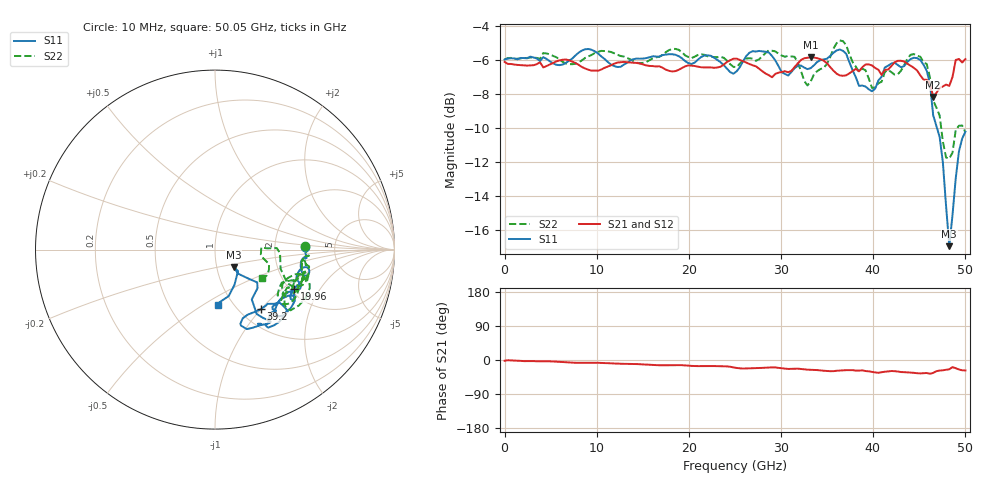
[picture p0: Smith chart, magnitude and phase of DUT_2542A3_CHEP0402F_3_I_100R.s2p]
! 11/3/2025 4:29:20 PM
! C:\MESURES\046-TRL-DUT-CHEP\0402\DUT-2542A3-CHEP0402F-3-I.S2P
! CHANNEL.1 Sparams
! TR.MEASUREMENT
! CORRECTED.DATA
! RF.CORRECTION: CAL.A: FULL.TWO.PORT.CALCAL.A: Port 1,4
! AVERAGING.OFF
! IF.BANDWIDTH: 500HZ
! SWEEPTYPE:  FREQ.SWEEP(Linear)
! Reference Plane Port Info
! PORT:  PORT1  PORT4
! DISTANCE:  0  m  0  m
! TIME:  0  s  0  s
! PHASE.OFFSET:  0  deg.  0  deg.
! LOSS:  0  dB  0  dB
! REF.LOSS:  0  dB  0  dB
! REF.FREQ:  0  Hz  0  Hz
! Power Info
! POWER:  -10  dBm  -10  dBm
! EFF.POWER:  -10  dBm  -10  dBm
! SOURCE.ATTEN:  0  dB  0  dB
! TEST.ATTEN:  0  dB  0  dB
! PORTZ: Port1:50 Port4:50
# GHZ S RI R 50
! FREQ.GHZ  S11RE  S11IM  S41RE  S41IM  S14RE  S14IM  S44RE  S44IM
!; PortSelection: Port_14 (1-->1,4-->4)
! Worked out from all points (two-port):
!   144 points, 10 MHz to 50.05 GHz, reference 50 ohm
!   highest |S21| = -5.84 dB at 33.26 GHz (marker M1); lowest = -8.2 dB at 46.55 GHz (marker M2)
!   |S21| within 3 dB of the highest: start of sweep to end of sweep
!   lowest |S11| = -17.0 dB at 48.3 GHz (marker M3), VSWR 1.33, Z = 60.3 - j11.9 ohm
!   |S11| at or under -10 dB: 46.96 GHz to end of sweep
!   |S22| runs from -11.8 to -4.8 dB; largest |S21 - S12| = 0.012
!   S11 on the Smith chart (normalised r, x): 10 MHz: 3.02, +0.13; 19.96 GHz: 2.10, -1.21; 39.2 GHz: 1.24, -1.00; 50.05 GHz: 0.85, -0.58
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0.01  0.5028 0.0166  0.4948 -0.0176  0.4956 -0.0177  0.5033 0.0175
8.4088  0.5152 -0.1433  0.4741 -0.0622  0.4731 -0.061  0.4934 -0.0843
14.008  0.4698 -0.1829  0.4843 -0.088  0.4838 -0.0865  0.494 -0.0589
16.8076  0.4618 -0.2236  0.4665 -0.1153  0.466 -0.1127  0.489 -0.1531
19.95715  0.4397 -0.2192  0.4676 -0.1231  0.467 -0.1246  0.4952 -0.1298
25.2064  0.3419 -0.3141  0.4728 -0.1809  0.4727 -0.1784  0.4307 -0.2076
28.7059  0.4457 -0.2819  0.4253 -0.1542  0.4266 -0.151  0.5057 -0.1765
32.2054  0.338 -0.3447  0.459 -0.203  0.4595 -0.2035  0.444 -0.1378
33.25525  0.3051 -0.3636  0.4592 -0.2223  0.4602 -0.2212  0.3723 -0.2222
33.6052  0.3021 -0.378  0.4568 -0.2267  0.4586 -0.2242  0.3828 -0.2451
35.7049  0.2968 -0.4346  0.4067 -0.2297  0.4066 -0.228  0.4212 -0.3384
37.1047  0.4009 -0.3362  0.4033 -0.204  0.4022 -0.2038  0.526 -0.177
39.2044  0.2548 -0.3325  0.4253 -0.2362  0.4232 -0.2343  0.436 -0.17
40.6042  0.1414 -0.4131  0.3904 -0.2604  0.3943 -0.2565  0.3496 -0.2475
42.004  0.2438 -0.4243  0.4202 -0.234  0.4224 -0.2345  0.4117 -0.2097
43.75375  0.2642 -0.4184  0.4111 -0.2647  0.4123 -0.2628  0.4053 -0.303
45.85345  0.2686 -0.3809  0.3622 -0.2469  0.3629 -0.2439  0.4406 -0.2095
46.55335  0.2049 -0.2774  0.3232 -0.2189  0.3267 -0.2142  0.3655 -0.108
47.6032  0.1906 -0.1636  0.3729 -0.1913  0.3749 -0.1872  0.2889 0.00692
48.3031  0.1038 -0.0966  0.3833 -0.1736  0.3842 -0.1704  0.2554 -0.028
49.35295  0.0762 -0.2589  0.4578 -0.2134  0.4579 -0.2125  0.3004 -0.1136
50.05285  0.0156 -0.3078  0.4476 -0.233  0.4505 -0.2244  0.262 -0.1603
